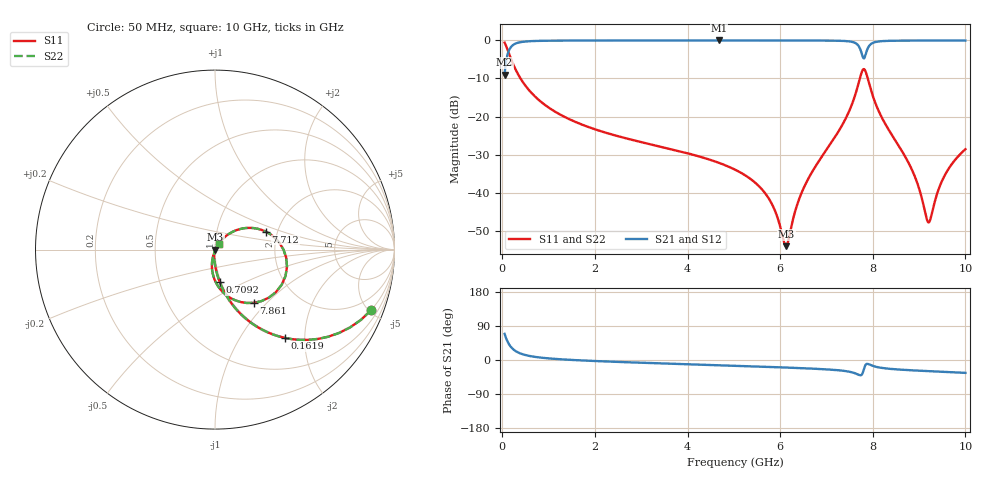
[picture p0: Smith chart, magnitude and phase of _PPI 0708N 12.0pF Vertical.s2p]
! S-Parameter data specifications (vertical orientation):
! Substrate: 40-mil Rogers 3003C, Substrate thickness, H=1.016mm, Dielectric constant, Er=3, Conductor thickness, T_mtl=0.043mm, Loss Tangent, Tand=0.003
! PCB Mounting Pad Footprint: Pad width, PadW=2.54mm , Pad length, PadL=0.51mm , Pad gap, PadG (edge-to-edge)=0.71mm , Reference planes=1.73mm apart
! Created Tue Jan 16 08:47:18 2018
# GHz S MA R 50
! 2 Port Network Data from SP1.SP block
! freq  magS11  angS11  magS21  angS21  magS12  angS12  magS22  angS22
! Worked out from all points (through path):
!   801 points, 50 MHz to 10 GHz, reference 50 ohm
!   highest |S21| = -0.02 dB at 4.677 GHz (marker M1); lowest = -9.0 dB at 50 MHz (marker M2)
!   group delay of S21, straight-line fit = 13 ps
!   lowest |S11| = -54.0 dB at 6.132 GHz (marker M3), VSWR 1.00, Z = 50.2 - j0.0632 ohm
!   |S11| at or under -10 dB: 393.8 MHz to 7.721 GHz (7.327 GHz wide, 181 % of centre); 7.891 GHz to end of sweep
!   |S22| runs from -54.0 to -0.6 dB; largest |S21 - S12| = 0
!   S11 on the Smith chart (normalised r, x): 50 MHz: 0.99, -5.20; 161.9 MHz: 0.99, -1.61; 709.2 MHz: 0.99, -0.37; 7.712 GHz: 1.74, +0.38; 7.861 GHz: 1.23, -0.84; 10 GHz: 1.05, +0.06
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0.05  0.9342 -21.1  0.3565 68.9  0.3565 68.9  0.9342 -21.1
0.1619375  0.629 -51.5  0.7772 38.4  0.7772 38.4  0.629 -51.5
0.3360625  0.3636 -69.7  0.9312 20.2  0.9312 20.2  0.3636 -69.7
0.7091875  0.1828 -81.7  0.9827 8.2  0.9827 8.2  0.1828 -81.7
1.716625  0.07868 -90.7  0.9962 -1.2  0.9962 -1.2  0.07868 -90.7
3.370812  0.0409 -97.4  0.998 -8.7  0.998 -8.7  0.0409 -97.4
4.67675  0.02474 -101.0  0.9982 -13.9  0.9982 -13.9  0.02474 -101.0
5.025  0.02013 -101.4  0.9982 -15.3  0.9982 -15.3  0.02013 -101.4
5.709062  0.009257 -97.7  0.998 -18.1  0.998 -18.1  0.009257 -97.7
6.131938  0.001993 -18.4  0.9977 -19.9  0.9977 -19.9  0.001993 -18.4
6.405563  0.008142 52.0  0.9973 -21.2  0.9973 -21.2  0.008142 52.0
6.691625  0.01885 58.1  0.9965 -22.8  0.9965 -22.8  0.01885 58.1
7.400563  0.09057 51.9  0.9815 -29.0  0.9815 -29.0  0.09057 51.9
7.7115  0.301 19.3  0.8115 -39.9  0.8115 -39.9  0.301 19.3
7.786125  0.4123 -13.4  0.6019 -33.1  0.6019 -33.1  0.4123 -13.4
7.86075  0.3666 -54.0  0.7005 -10.8  0.7005 -10.8  0.3666 -54.0
7.997562  0.1895 -87.5  0.9252 -15.4  0.9252 -15.4  0.1895 -87.5
8.345812  0.06675 -103.7  0.9867 -23.0  0.9867 -23.0  0.06675 -103.7
8.868187  0.0187 -102.3  0.9946 -27.4  0.9946 -27.4  0.0187 -102.3
9.204  0.00408 -28.7  0.9955 -29.4  0.9955 -29.4  0.00408 -28.7
9.55225  0.01686 45.5  0.9956 -31.4  0.9956 -31.4  0.01686 45.5
10  0.03734 50.1  0.995 -33.9  0.995 -33.9  0.03734 50.1
